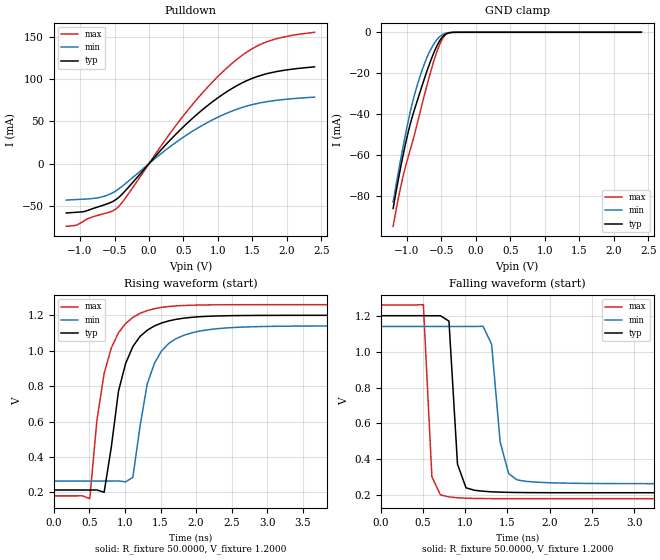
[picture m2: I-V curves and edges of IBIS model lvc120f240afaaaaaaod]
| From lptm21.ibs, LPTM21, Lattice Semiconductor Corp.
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|   Model lvc120f240afaaaaaaod
[Model]   lvc120f240afaaaaaaod
Model_type   I/O_open_drain
Polarity   Non-Inverting
Enable   Active-Low
Vinl =   0.4200V
Vinh =   0.7800V
Vmeas =   0.6000V
Cref =   0.0F
Rref =   1.0000M
Vref =   0.0V
C_comp   4.2000pF   3.8000pF   7.5000pF
[Temperature Range]   25.0000   0.1050k   -40.0000
[Voltage Range]   1.2000V   1.1400V   1.2600V
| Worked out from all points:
|   slope of the pulldown table from 0 to 0.18 V, typ, clamps not added: 10.8 ohm
|   GND clamp passes 1 mA (typ) near -0.44 V on its own axis
|   rising waveform, R_fixture 50.0000, V_fixture 1.2000: 20-80 % time 299ps typ, 300ps min, 284ps max; typ from 0.214 V to 1.2 V
|   falling waveform, R_fixture 50.0000, V_fixture 1.2000: 20-80 % time 75ps typ, 120ps min, 68.3ps max; typ from 1.2 V to 0.214 V
[Pulldown]
|Voltage   I(typ)   I(min)   I(max)
-1.2V     -58.19mA   -42.94mA   -73.91mA
-1.04V    -57.28mA   -42.27mA   -72.04mA
-720mV    -50.52mA   -39.95mA   -60.48mA
-520mV    -44.42mA   -34.08mA   -55.51mA
-440mV    -39.92mA   -29.91mA   -50.64mA
200mV     18.48mA    13.43mA    23.8mA
560mV     48.15mA    34.55mA    62.73mA
920mV     72.93mA    51.6mA     96.24mA
1.28V     92.25mA    64.33mA    123.4mA
1.48V     100.1mA    69.3mA     134.8mA
1.72V     106.4mA    73.26mA    144.1mA
2.4V      114.2mA    78.47mA    155mA
[GND_clamp]
|Voltage   I(typ)   I(min)   I(max)
-1.2V     -86.19mA   -82.94mA   -94.91mA
-1.1V     -67.71mA   -63.95mA   -77.28mA
-1V       -51.52mA   -46.57mA   -63.21mA
-920mV    -41.11mA   -34.53mA   -53.74mA
-840mV    -32.47mA   -24.81mA   -43.38mA
-740mV    -22.05mA   -14.9mA    -29.96mA
-640mV    -12.58mA   -7.515mA   -17.52mA
-580mV    -7.752mA   -4.29mA    -10.99mA
-520mV    -3.927mA   -2.008mA   -5.609mA
-440mV    -951.3uA   -477uA     -1.256mA
-300mV    -18.83uA   -15.98uA   -16.74uA
2.4V      0A         0A         0A
[Ramp]
| variable   typ   min   max
dV/dt_r  0.5916/0.2957n   0.5253/0.2972n   0.6474/0.2808n
dV/dt_f  0.5916/74.2487p   0.5253/0.1184n   0.6475/67.5768p
R_load = 50.0000
[Rising Waveform]
R_fixture=   50.0000
V_fixture=   1.2000
V_fixture_min=   1.1400
V_fixture_max=   1.2600
|time   V(typ)   V(min)   V(max)
0s        214mV      264.5mV    180.9mV
505.1ps   213.9mV    264.5mV    165.1mV
606.1ps   214.4mV    264.5mV    608.2mV
707.1ps   201.1mV    264.5mV    871.8mV
909.1ps   772.3mV    264.9mV    1.102V
1.111ns   1.024V     285.6mV    1.188V
1.313ns   1.116V     812.8mV    1.227V
1.616ns   1.168V     1.041V     1.25V
2.323ns   1.196V     1.125V     1.259V
10ns      1.2V       1.14V      1.26V
[Falling Waveform]
R_fixture=   50.0000
V_fixture=   1.2000
V_fixture_min=   1.1400
V_fixture_max=   1.2600
|time   V(typ)   V(min)   V(max)
0s        1.2V       1.14V      1.26V
505.1ps   1.2V       1.14V      1.261V
606.1ps   1.2V       1.14V      303.3mV
808.1ps   1.17V      1.14V      190.8mV
909.1ps   372.9mV    1.14V      185.9mV
1.111ns   227.6mV    1.14V      182.2mV
1.313ns   219.1mV    1.04V      181.2mV
1.414ns   217.3mV    496.9mV    181.1mV
1.616ns   215.3mV    285.4mV    180.9mV
10ns      214mV      264.5mV    180.9mV
